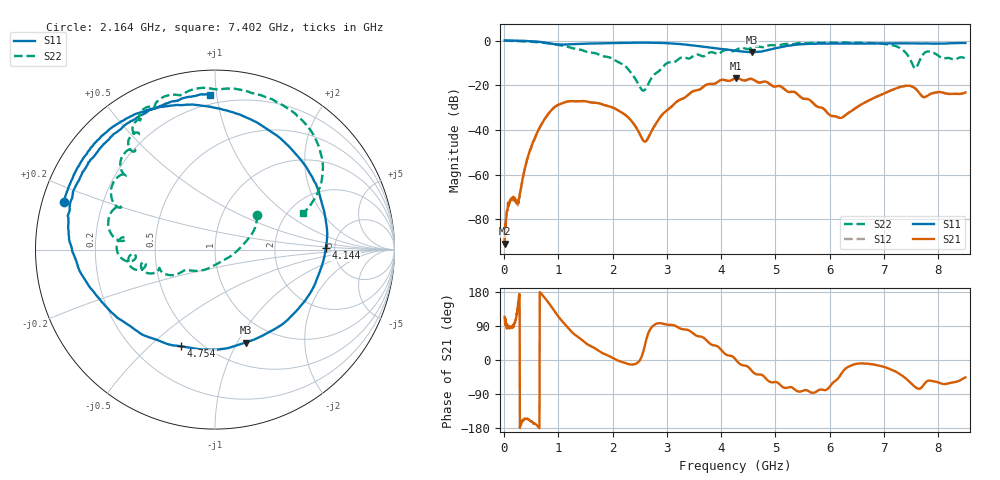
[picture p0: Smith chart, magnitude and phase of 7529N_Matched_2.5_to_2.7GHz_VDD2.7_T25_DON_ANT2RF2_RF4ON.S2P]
!Agilent Technologies,E5071C,MY46417908,A.11.23
!Date: Wed Oct 16 15:59:26 2019
!Data & Calibration Information:
!Freq	S11:SOLT2(ON)	S21:SOLT2(ON)	S12:SOLT2(ON)	S22:SOLT2(ON)
!PortZ  Port1:50+j0  Port2:50+j0
!Above PortZ is port z conversion or system Z0 setting when saving the data.
!When reading, reference impedance value at option line is always used.
# Hz S dB R 50
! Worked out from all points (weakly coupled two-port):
!   1601 points, 10 MHz to 8.5 GHz, reference 50 ohm
!   highest |S21| = -16.85 dB at 4.276 GHz (marker M1); lowest = -91.0 dB at 10 MHz (marker M2)
!   lowest |S11| = -5.3 dB at 4.568 GHz (marker M3), VSWR 3.40, Z = 36.8 - j54.2 ohm
!   |S11| at or under -10 dB: nowhere
!   |S22| runs from -22.4 to 0.0 dB; largest |S21 - S12| = 0.0013
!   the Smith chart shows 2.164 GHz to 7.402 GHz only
!   S11 on the Smith chart (normalised r, x): 2.164 GHz: 0.06, +0.15; 4.144 GHz: 4.22, +0.11; 4.754 GHz: 0.40, -0.63; 7.402 GHz: 0.14, +0.96
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1e7  0.01 178.8  -90.97 113.8  -92.05 157.4  -0.05 179.0
2.647e8  -0.09 148.0  -72.86 156.6  -72.78 154.6  -0.30 165.2
5.83075e8  -0.44 95.7  -42.78 -169.6  -42.84 -169.2  -0.69 147.9
8.855312e8  -1.48 8.0  -30.83 138.2  -30.81 138.4  -1.44 130.0
1.124312e9  -1.78 -67.1  -27.60 93.8  -27.59 93.7  -2.46 114.6
1.426769e9  -1.47 -124.1  -27.12 54.0  -27.12 53.8  -4.21 93.8
2.164338e9  -1.08 162.4  -32.16 -4.7  -32.19 -5.0  -10.34 39.8
2.588838e9  -0.97 138.0  -45.22 35.5  -45.24 35.5  -22.21 -74.6
2.843538e9  -1.06 126.5  -35.51 97.1  -35.53 96.9  -13.86 -145.6
3.543962e9  -2.39 77.9  -22.33 64.2  -22.36 64.0  -6.27 -170.9
4.143569e9  -4.20 0.8  -18.08 11.8  -18.11 11.7  -4.38 157.7
4.255e9  -4.57 -16.2  -16.95 3.3  -16.96 3.2  -4.52 156.4
4.276225e9  -4.60 -19.5  -16.85 -0.3  -16.86 -0.6  -4.21 155.6
4.568069e9  -5.27 -71.8  -17.26 -29.2  -17.24 -29.4  -3.15 139.0
4.753788e9  -4.87 -109.2  -18.59 -39.6  -18.56 -39.8  -3.01 129.0
5.167675e9  -2.60 -166.3  -21.85 -73.5  -21.80 -73.7  -1.57 122.5
5.671769e9  -1.44 162.6  -27.49 -86.4  -27.42 -86.4  -1.02 110.7
6.202394e9  -1.38 136.1  -34.69 -38.7  -34.67 -38.9  -0.92 85.2
7.088538e9  -1.28 100.1  -22.70 -22.8  -22.74 -22.6  -1.77 44.9
7.401606e9  -1.28 91.7  -20.28 -48.5  -20.29 -48.9  -5.47 22.5
7.640388e9  -1.34 84.1  -23.16 -75.9  -23.13 -76.1  -9.88 74.0
8.5e9  -1.11 49.3  -23.26 -45.9  -23.29 -46.2  -8.10 46.9
